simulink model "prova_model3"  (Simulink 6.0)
settings: Solver=ode45  StartTime=0.0  StopTime=T  RelTol=1e-3
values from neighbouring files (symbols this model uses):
  Tc = 0.01    [createsimulation.m]    (also in esercizio_riassuntivo_script1.m = 0.1)

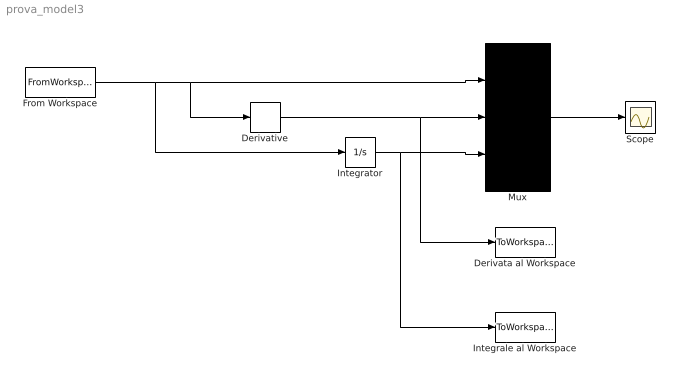
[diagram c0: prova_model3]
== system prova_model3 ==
  Derivata al Workspace : ToWorkspace  VariableName=dy  SampleTime=Tc  SaveFormat=Array
  Derivative : Derivative
  From Workspace : FromWorkspace  VariableName=[t y]  SampleTime=Tc
  Integrale al Workspace : ToWorkspace  VariableName=inty  SampleTime=Tc  SaveFormat=Array
  Integrator : Integrator
  Mux : Mux  Inputs=3
  Scope : Scope
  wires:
  From Workspace/1 -> Derivative/1, Mux/1, Integrator/1
  Derivative/1 -> Mux/2, Derivata al Workspace/1
  Integrator/1 -> Mux/3, Integrale al Workspace/1
  Mux/1 -> Scope/1
